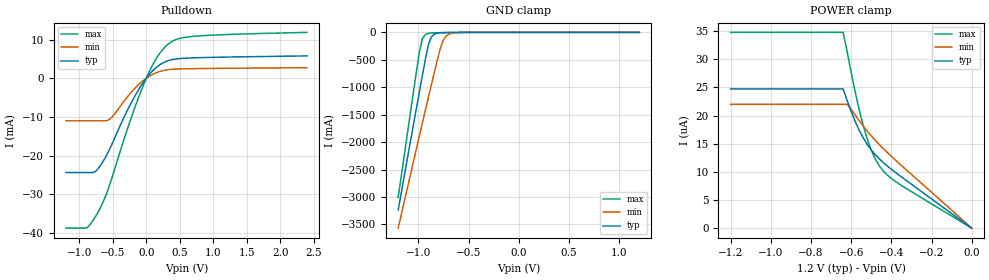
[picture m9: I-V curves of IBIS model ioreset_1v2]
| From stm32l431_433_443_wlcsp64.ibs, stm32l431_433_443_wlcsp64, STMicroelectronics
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|   Model ioreset_1v2
[Model]  ioreset_1v2
Model_type I/O_open_drain
Polarity   Inverting
Enable   Active-High
Vinl =   0.360000V
Vinh =   0.840000V
Vmeas =  0.600000V
Cref =   100.000000nF
Rref =   1.000000k
Vref =   1.200000V
C_comp   0.478720pF   0.386870pF   0.488870pF
[Temperature Range]   25.000000   0.125000k   -40.000000
[Pullup Reference]   1.200000V   1.080000V   1.320000V
[Pulldown Reference]   0.0V   0.0V   0.0V
[POWER Clamp Reference]   1.200000V   1.080000V   1.320000V
[GND Clamp Reference]   0.0V   0.0V   0.0V
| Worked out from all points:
|   slope of the pulldown table from 0 to 0.18 V, typ, clamps not added: 55.8 ohm
|   GND clamp passes 1 mA (typ) near -0.60 V on its own axis
[Pulldown]
|Voltage   I(typ)   I(min)   I(max)
-1.2V     -24.41mA   -11.01mA   -38.83mA
-880mV    -24.41mA   -11.01mA   -38.66mA
-720mV    -23.44mA   -11.01mA   -34.71mA
-600mV    -20.17mA   -11.01mA   -30.21mA
-520mV    -17.35mA   -10.18mA   -26.2mA
-240mV    -6.83mA    -3.923mA   -10.98mA
-40mV     -934.1uA   -487.3uA   -1.63mA
120mV     2.392mA    1.255mA    4.286mA
320mV     4.57mA     2.255mA    8.784mA
480mV     5.107mA    2.449mA    10.28mA
720mV     5.336mA    2.535mA    10.93mA
2.4V      5.832mA    2.779mA    11.93mA
[GND_clamp]
|Voltage   I(typ)   I(min)   I(max)
-1.2V     -3.237A    -3.567A    -3.007A
-990mV    -1.09A     -1.891A    -366.7mA
-960mV    -790.4mA   -1.655A    -117.3mA
-930mV    -495.2mA   -1.419A    -39.03mA
-900mV    -224mA     -1.186A    -17.33mA
-870mV    -83.94mA   -954.7mA   -11.02mA
-780mV    -7.786mA   -289.5mA   -5.907mA
-750mV    -4.95mA    -134.8mA   -4.824mA
-720mV    -3.507mA   -62.23mA   -3.833mA
-660mV    -1.911mA   -14.46mA   -2.15mA
-540mV    -364.7uA   -1.228mA   -309.9uA
1.2V      0A         0A         0A
[POWER_clamp]
|Voltage   I(typ)   I(min)   I(max)
-1.2V     24.72uA    21.98uA    34.76uA
-640mV    24.72uA    21.98uA    34.76uA
-620mV    22.7uA     21.98uA    31.37uA
-580mV    18.97uA    20.1uA     24.2uA
-560mV    17.4uA     19.1uA     21.04uA
-540mV    16.05uA    18.14uA    18.24uA
-520mV    14.89uA    17.24uA    15.84uA
-500mV    13.9uA     16.4uA     13.86uA
-460mV    12.31uA    14.85uA    11.08uA
-420mV    11.04uA    13.44uA    9.427uA
-380mV    9.91uA     12.11uA    8.305uA
0V        0A         0A         0A
[Ramp]
| variable   typ   min   max
dV/dt_r  0.71922/0.60515u   0.64668/0.60033u   0.79151/0.60018u
dV/dt_f  0.71922/37.88688n   0.64668/77.76066n   0.79151/22.19591n
R_load = 40.000000k
